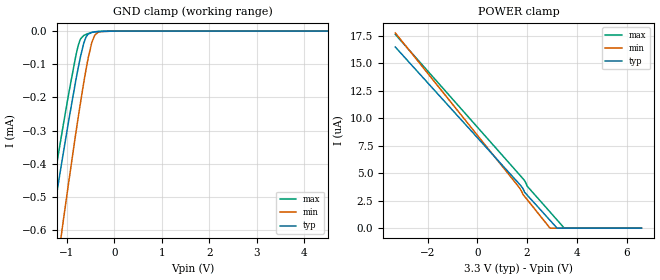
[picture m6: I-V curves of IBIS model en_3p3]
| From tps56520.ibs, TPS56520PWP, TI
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|   en_3p3 Model
[Model]   en_3p3
Model_type   Input
Vinl = 0.6
Vinh = 1.8
|   typ   min   max
|   (nom PVT)   (fast PVT)   (slow PVT)
C_comp   4.606e-12   4.365e-12   4.780e-12
| Where nom  PVT is Nominal Process, 3.3V, 27C
|   Fast PVT is Strong Process,  3.6V, -40C
|   Slow PVT is Weak Process,   3V, 125C
[Voltage Range]   3.3   3   3.6
|Junction Temperature
[Temperature Range]   27   125   -40
[Power Clamp Reference]   3.3   3   3.6
[GND Clamp Reference]   0   0   0
[GND Clamp]
|   Voltage   I(typ)   I(min)   I(max)
-3.3V     -2.599mA   -3.237mA   -2.406mA
-1.452V   -711.8uA   -978.7uA   -614uA
-1.32V    -589.8uA   -834.6uA   -496.9uA
-1.089V   -382.7uA   -589.7uA   -297.3uA
-953.7mV  -266.6uA   -451.3uA   -185.3uA
-754.8mV  -108.6uA   -257.5uA   -42.35uA
-643.5mV  -37.68uA   -157.5uA   -13.52uA
-585.6mV  -15.85uA   -109.9uA   -9.561uA
-471mV    -4.193uA   -34.3uA    -3.828uA
-408mV    -2.325uA   -11.93uA   -2.073uA
-279mV    -980.7nA   -1.517uA   -978.7nA
6.6V      0A         0A         0A
[POWER Clamp]
|   Voltage   I(typ)   I(min)   I(max)
-3.3V     16.47uA    17.75uA    17.62uA
1.617V    4.193uA    3.889uA    5.056uA
1.812V    3.671uA    3.194uA    4.558uA
1.927V    3.2uA      2.811uA    4.212uA
1.999V    3.021uA    2.608uA    3.833uA
2.922V    715.5nA    0A         1.475uA
3.208V    0A         0A         744.3nA
3.497V    0A         0A         0A
6.6V      0A         0A         0A
